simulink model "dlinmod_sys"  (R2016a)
settings: Solver=FixedStepAuto  StartTime=0.0  StopTime=10  FixedStep=0.001  RelTol=1e-6  AbsTol=1e-6

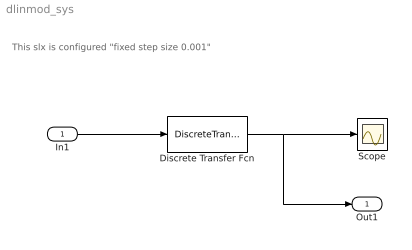
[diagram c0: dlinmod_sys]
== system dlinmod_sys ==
  note: This slx is configured "fixed step size 0.001"
  In1 : Inport
  Discrete Transfer Fcn : DiscreteTransferFcn  Numerator=1*(1-0.98)  Denominator=[1 -0.98]
  Scope : Scope
  Out1 : Outport
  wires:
  Discrete Transfer Fcn/1 -> Out1/1, Scope/1
  In1/1 -> Discrete Transfer Fcn/1
